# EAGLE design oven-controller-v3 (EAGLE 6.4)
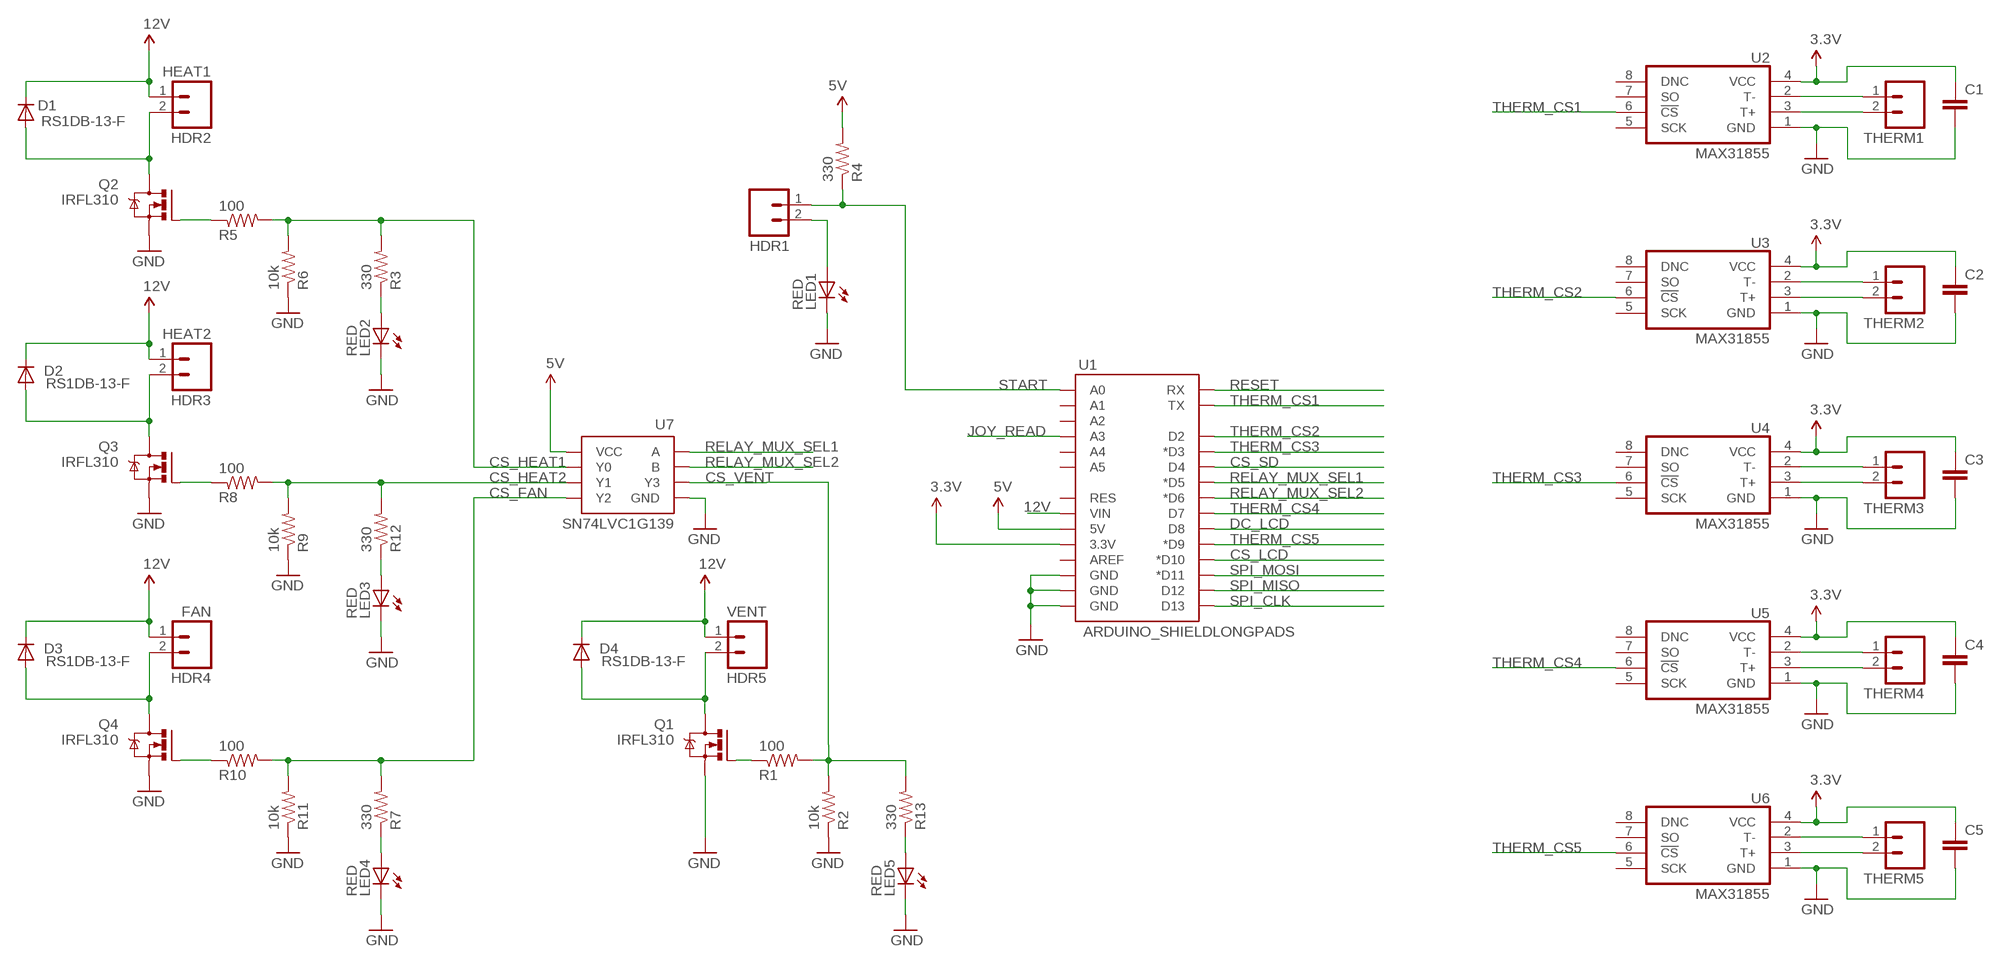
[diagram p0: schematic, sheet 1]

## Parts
C1  C-EUC0603K  [C0603K]
C2  C-EUC0603K  [C0603K]
C3  C-EUC0603K  [C0603K]
C4  C-EUC0603K  [C0603K]
C5  C-EUC0603K  [C0603K]
D1  RS1DB-13-F  DIODESMA-ALT  [SMA-DIODE_ALT]
D2  RS1DB-13-F  DIODESMA-ALT  [SMA-DIODE_ALT]
D3  RS1DB-13-F  DIODESMA-ALT  [SMA-DIODE_ALT]
D4  RS1DB-13-F  DIODESMA-ALT  [SMA-DIODE_ALT]
HDR1  M023.5MM_LOCK  [SCREWTERMINAL-3.5MM-2_LOCK]
HDR2  HEAT1  M023.5MM_LOCK  [SCREWTERMINAL-3.5MM-2_LOCK]
HDR3  HEAT2  M023.5MM_LOCK  [SCREWTERMINAL-3.5MM-2_LOCK]
HDR4  FAN  M023.5MM_LOCK  [SCREWTERMINAL-3.5MM-2_LOCK]
HDR5  VENT  M023.5MM_LOCK  [SCREWTERMINAL-3.5MM-2_LOCK]
LED1  RED  LED0603  [LED-0603]
LED2  RED  LED0603  [LED-0603]
LED3  RED  LED0603  [LED-0603]
LED4  RED  LED0603  [LED-0603]
LED5  RED  LED0603  [LED-0603]
Q1  IRFL310  IRF520  [TO220BV]
Q2  IRFL310  IRF520  [TO220BV]
Q3  IRFL310  IRF520  [TO220BV]
Q4  IRFL310  IRF520  [TO220BV]
R1  100  R-US_0603-C-NOSILK  [0603-C-NOSILK]
R2  10k  R-US_0603-C-NOSILK  [0603-C-NOSILK]
R3  330  R-US_0603-C-NOSILK  [0603-C-NOSILK]
R4  330  R-US_0603-C-NOSILK  [0603-C-NOSILK]
R5  100  R-US_0603-C-NOSILK  [0603-C-NOSILK]
R6  10k  R-US_0603-C-NOSILK  [0603-C-NOSILK]
R7  330  R-US_0603-C-NOSILK  [0603-C-NOSILK]
R8  100  R-US_0603-C-NOSILK  [0603-C-NOSILK]
R9  10k  R-US_0603-C-NOSILK  [0603-C-NOSILK]
R10  100  R-US_0603-C-NOSILK  [0603-C-NOSILK]
R11  10k  R-US_0603-C-NOSILK  [0603-C-NOSILK]
R12  330  R-US_0603-C-NOSILK  [0603-C-NOSILK]
R13  330  R-US_0603-C-NOSILK  [0603-C-NOSILK]
THERM1  M023.5MM_LOCK  [SCREWTERMINAL-3.5MM-2_LOCK]
THERM2  M023.5MM_LOCK  [SCREWTERMINAL-3.5MM-2_LOCK]
THERM3  M023.5MM_LOCK  [SCREWTERMINAL-3.5MM-2_LOCK]
THERM4  M023.5MM_LOCK  [SCREWTERMINAL-3.5MM-2_LOCK]
THERM5  M023.5MM_LOCK  [SCREWTERMINAL-3.5MM-2_LOCK]
U1  ARDUINO_SHIELDLONGPADS  [DUEMILANOVE_SHIELD_LONGPADS]
U2  MAX31855  IC_MAX31855-SO-8  [SO-8]
U3  MAX31855  IC_MAX31855-SO-8  [SO-8]
U4  MAX31855  IC_MAX31855-SO-8  [SO-8]
U5  MAX31855  IC_MAX31855-SO-8  [SO-8]
U6  MAX31855  IC_MAX31855-SO-8  [SO-8]
U7  SN74LVC1G139  [8LSSOP]

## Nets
3.3V: C1.1 C2.1 C3.1 C4.1 C5.1 U1.3.3V U2.4(VCC) U3.4(VCC) U4.4(VCC) U5.4(VCC) U6.4(VCC)
5V: R4.2 U1.5V U7.P$8(VCC)
12V: D1.C D2.C D3.C D4.C HDR2.1 HDR3.1 HDR4.1 HDR5.1 U1.VIN
CS_FAN: R7.2 R10.2 R11.2 U7.P$5(Y2)
CS_HEAT1: R3.2 R5.2 R6.2 U7.P$7(Y0)
CS_HEAT2: R8.2 R9.2 R12.2 U7.P$6(Y1)
CS_LCD: U1.D10(*D10)
CS_SD: U1.D4
CS_VENT: R1.2 R2.2 R13.2 U7.P$3(Y3)
DC_LCD: U1.D8
GND: C1.2 C2.2 C3.2 C4.2 C5.2 LED1.C LED2.C LED3.C LED4.C LED5.C Q1.S Q2.S Q3.S Q4.S R2.1 R6.1 R9.1 R11.1 U1.GND@0(GND) U1.GND@1(GND) U1.GND@2(GND) U2.1(GND) U3.1(GND) U4.1(GND) U5.1(GND) U6.1(GND) U7.P$4(GND)
HDR3: D3.A HDR4.2 Q4.D
JOY_READ: U1.A3
N$1: Q2.G R5.1
N$2: Q1.G R1.1
N$3: D4.A HDR5.2 Q1.D
N$4: D1.A HDR2.2 Q2.D
N$5: THERM1.1 U2.2(T-)
N$6: THERM1.2 U2.3(T+)
N$7: LED2.A R3.1
N$8: THERM2.1 U3.2(T-)
N$9: LED4.A R7.1
N$10: HDR1.2 LED1.A
N$11: THERM2.2 U3.3(T+)
N$12: THERM3.1 U4.2(T-)
N$13: THERM3.2 U4.3(T+)
N$14: THERM4.1 U5.2(T-)
N$15: THERM4.2 U5.3(T+)
N$16: THERM5.1 U6.2(T-)
N$17: THERM5.2 U6.3(T+)
N$18: LED3.A R12.1
N$19: LED5.A R13.1
N$20: Q3.G R8.1
N$21: D2.A HDR3.2 Q3.D
N$23: Q4.G R10.1
RELAY_MUX_SEL1: U1.D5(*D5) U7.P$1(A)
RELAY_MUX_SEL2: U1.D6(*D6) U7.P$2(B)
RESET: U1.RX
SPI_CLK: U1.D13
SPI_MISO: U1.D12
SPI_MOSI: U1.D11(*D11)
START: HDR1.1 R4.1 U1.A0
THERM_CS1: U1.TX U2.6(!CS)
THERM_CS2: U1.D2 U3.6(!CS)
THERM_CS3: U1.D3(*D3) U4.6(!CS)
THERM_CS4: U1.D7 U5.6(!CS)
THERM_CS5: U1.D9(*D9) U6.6(!CS)
Unconnected: U1.A1 U1.A2 U1.A4 U1.A5 U1.AREF U1.RES U2.5(SCK) U2.7(SO) U2.8(DNC) U3.5(SCK) U3.7(SO) U3.8(DNC) U4.5(SCK) U4.7(SO) U4.8(DNC) U5.5(SCK) U5.7(SO) U5.8(DNC) U6.5(SCK) U6.7(SO) U6.8(DNC)

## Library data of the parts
C1-C5 = rcl_custom:C-EU: CAPACITOR, European symbol
D1-D4 = SparkFun-DiscreteSemi:DIODE: Diode
HDR1-HDR5 THERM1-THERM5 = SparkFun-Connectors:M02: Header 2
LED1-LED5 = SparkFun-LED:LED: LEDs
Q1-Q4 = transistor-power:IRF520: HEXFET Power MOSFET
R1-R13 = rcl_custom:R-US_: RESISTOR, American symbol
U1 = SparkFun-Boards:ARDUINO_SHIELD: Arduino shield footprint
U2-U6 = dp_devices:IC_MAX31855
U7 = wicker:SN74LVC1G139

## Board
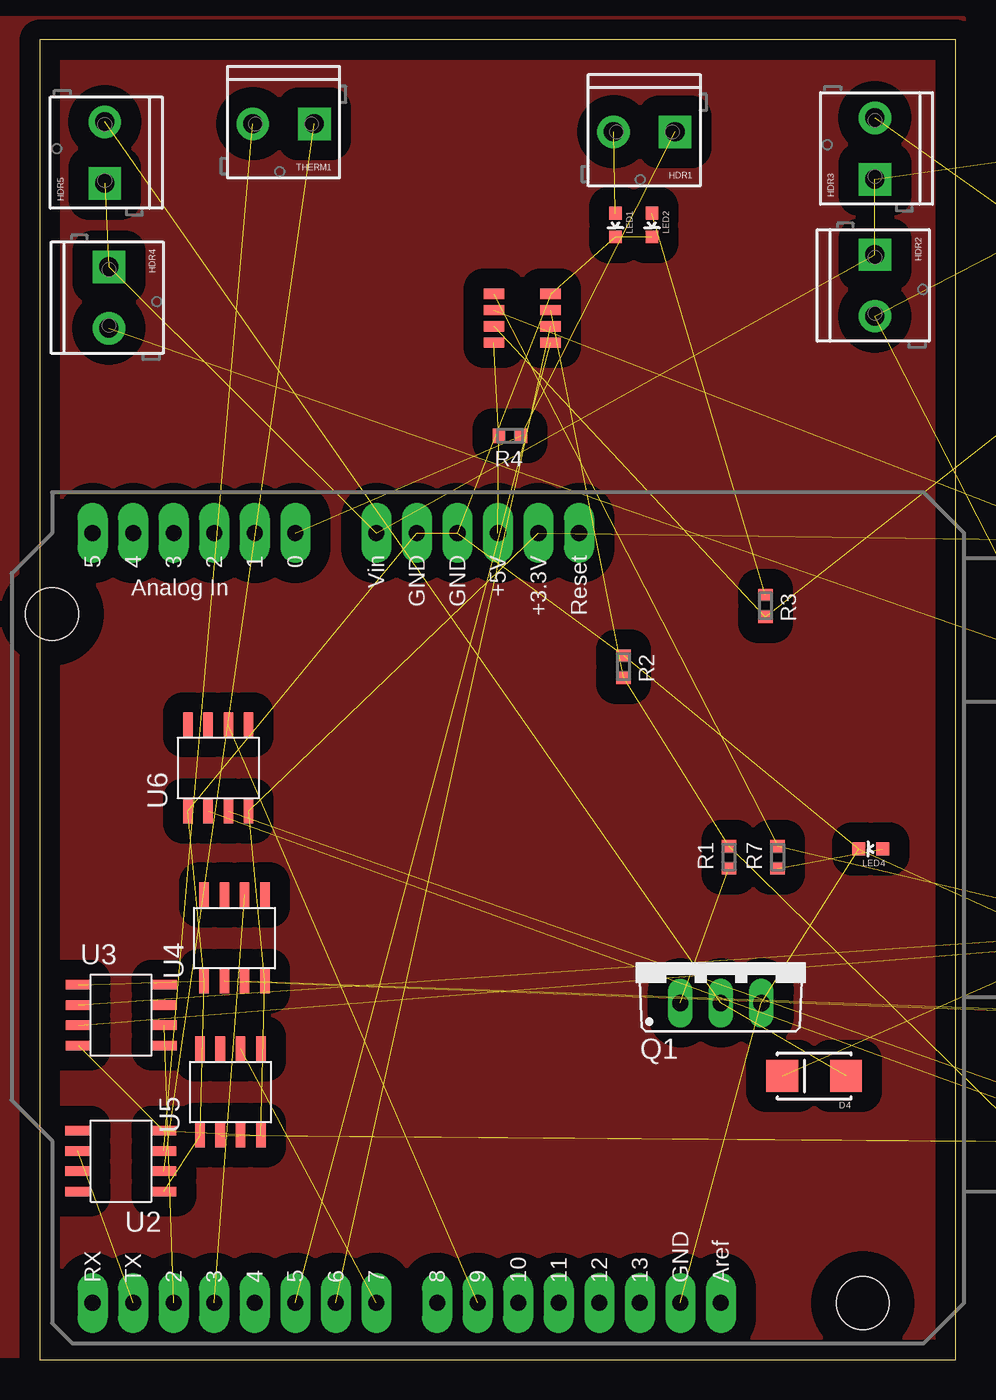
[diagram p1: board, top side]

Size 57.38 x 82.73 mm. Coordinates in mm from the lower left corner, seen from the top.
Outline: 0,0 57.38,0 57.38,82.73 0,82.73 0,0
Copper layers (1*16): Top 0.0178mm / dielectric 59mil / Bottom 0.0178mm
Design rules "epl-lpkf": minimum track width 8mil, minimum drill 0.35mm, track to track 8mil, track to pad 8mil, pad to pad 8mil, via to via 8mil, smd to smd 8mil, copper to edge 15mil, drill to drill 15mil, minimum pad ring 8mil, minimum via ring 8mil, stop-mask expansion 3mil, vias tented up to drill 0mil, thermal gap 10mil

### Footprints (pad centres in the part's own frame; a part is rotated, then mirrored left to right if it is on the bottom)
C0603K = smd 1.05 x 1.08: 1 -0.875,0; 2 0.875,0
SMA-DIODE_ALT = smd 2 x 2: A -2,0; C 2,0
SCREWTERMINAL-3.5MM-2_LOCK = drill 1.2 pad 2.032 square: 1 -0.178,0 | drill 1.2 pad 2.032: 2 3.678,0
LED-0603 = smd 0.8 x 0.8: A 0,-0.75; C 0,0.75
TO220BV = drill 1.016 long: D 0,-2.54; G -2.54,-2.54; S 2.54,-2.54
0603-C-NOSILK = smd 0.75 x 0.9: 1 -0.7,0; 2 0.7,0
DUEMILANOVE_SHIELD_LONGPADS = drill 1.016 pad 1.88 long: 3.3V 50.8,26.67; 5V 50.8,29.21; A0 50.8,41.91; A1 50.8,44.45; A2 50.8,46.99; A3 50.8,49.53; A4 50.8,52.07; A5 50.8,54.61; AREF 2.54,15.24; D2 2.54,49.53; D3 2.54,46.99; D4 2.54,44.45; D5 2.54,41.91; D6 2.54,39.37; D7 2.54,36.83; D8 2.54,33.02; D9 2.54,30.48; D10 2.54,27.94; D11 2.54,25.4; D12 2.54,22.86; D13 2.54,20.32; GND@0 50.8,31.75; GND@1 50.8,34.29; GND@2 2.54,17.78; RES 50.8,24.13; RX 2.54,54.61; TX 2.54,52.07; VIN 50.8,36.83 | hole 3.302: 45.72,57.15; 2.54,6.35
SO-8 = smd 0.6 x 1.55: 1 -1.905,-2.69; 2 -0.635,-2.69; 3 0.635,-2.69; 4 1.905,-2.69; 5 1.905,2.71; 6 0.635,2.71; 7 -0.635,2.71; 8 -1.905,2.71
8LSSOP = smd 1.27 x 0.635: P$1 -1.778,2.794; P$2 -1.778,1.778; P$3 -1.778,0.762; P$4 -1.778,-0.254; P$5 1.778,-0.254; P$6 1.778,0.762; P$7 1.778,1.778; P$8 1.778,2.794

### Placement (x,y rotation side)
C1  not placed on the board
C2  not placed on the board
C3  not placed on the board
C4  not placed on the board
C5  not placed on the board
D1  not placed on the board
D2  not placed on the board
D3  not placed on the board
D4  48.51,17.78 180 top
HDR1  39.62,76.96 180 top
HDR2  52.32,69.09 270 top
HDR3  52.32,74.17 90 top
HDR4  4.32,68.33 270 top
HDR5  4.06,73.91 90 top
LED1  36.07,71.12 180 top
LED2  38.35,71.12 180 top
LED3  not placed on the board
LED4  52.07,32 90 top
LED5  not placed on the board
Q1  42.67,24.89 0 top
Q2  not placed on the board
Q3  not placed on the board
Q4  not placed on the board
R1  43.18,31.5 90 top
R2  36.58,43.43 270 top
R3  45.47,47.24 270 top
R4  29.46,57.91 180 top
R5  not placed on the board
R6  not placed on the board
R7  46.23,31.5 90 top
R8  not placed on the board
R9  not placed on the board
R10  not placed on the board
R11  not placed on the board
R12  not placed on the board
R13  not placed on the board
THERM1  17.02,77.47 180 top
THERM2  not placed on the board
THERM3  not placed on the board
THERM4  not placed on the board
THERM5  not placed on the board
U1  57.91,1.02 90 top
U2  5.08,12.45 90 top
U3  5.08,21.59 270 top
U4  12.19,26.42 0 top
U5  11.94,16.76 0 top
U6  11.18,37.08 0 top
U7  30.23,66.55 180 top

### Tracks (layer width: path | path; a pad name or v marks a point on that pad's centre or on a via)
3.3V  (10 unrouted)
5V  (2 unrouted)
12V  (8 unrouted)
CS_FAN  (3 unrouted)
CS_HEAT1  (3 unrouted)
CS_HEAT2  (3 unrouted)
CS_VENT  (3 unrouted)
GND  (26 unrouted)
HDR3  (2 unrouted)
N$1  (1 unrouted)
N$2  (1 unrouted)
N$3  (2 unrouted)
N$4  (2 unrouted)
N$5  (1 unrouted)
N$6  (1 unrouted)
N$7  (1 unrouted)
N$8  (1 unrouted)
N$9  (1 unrouted)
N$10  (1 unrouted)
N$11  (1 unrouted)
N$12  (1 unrouted)
N$13  (1 unrouted)
N$14  (1 unrouted)
N$15  (1 unrouted)
N$16  (1 unrouted)
N$17  (1 unrouted)
N$18  (1 unrouted)
N$19  (1 unrouted)
N$20  (1 unrouted)
N$21  (2 unrouted)
N$22
  pour Top (isolate 1.27): -4.83,84.07 -4.83,0.25 57.91,0.25 57.91,84.07
N$23  (1 unrouted)
RELAY_MUX_SEL1  (1 unrouted)
RELAY_MUX_SEL2  (1 unrouted)
START  (2 unrouted)
THERM_CS1  (1 unrouted)
THERM_CS2  (1 unrouted)
THERM_CS3  (1 unrouted)
THERM_CS4  (1 unrouted)
THERM_CS5  (1 unrouted)

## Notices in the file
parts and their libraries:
SparkFun-Boards: Licensing: CC v3.0 Share-Alike You are welcome to use this library for commercial purposes.
